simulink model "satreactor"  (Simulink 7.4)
settings: Solver=ode15s  StartTime=0.0  StopTime=0.05  MaxStep=1e-4  RelTol=1e-7  AbsTol=1e-7
libraries: simulink x1

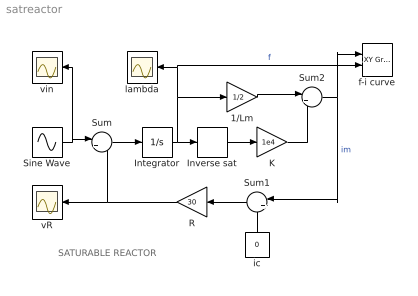
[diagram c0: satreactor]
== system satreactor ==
  note: SATURABLE REACTOR
  1/Lm : Gain  Gain=1/2  ParameterDataType=sfix(16)  ParameterScaling=2^0  OutDataType=sfix(16)  OutScaling=2^0
  Integrator : Integrator
  Inverse sat : DeadZone  LowerValue=-.25  UpperValue=.25
  K : Gain  Gain=1e4  ParameterDataType=sfix(16)  ParameterScaling=2^0  OutDataType=sfix(16)  OutScaling=2^0
  R : Gain  Gain=30  ParameterDataType=sfix(16)  ParameterScaling=2^0  OutDataType=sfix(16)  OutScaling=2^0
  Sine Wave : Sin  Amplitude=120*sqrt(2)  Bias=0  Frequency=2*pi*60  Phase=0  Samples=10  SampleTime=0
  Sum : Sum  Inputs=|+-  OutDataType=sfix(16)  OutScaling=2^0
  Sum1 : Sum  Inputs=|+-  OutDataType=sfix(16)  OutScaling=2^0
  Sum2 : Sum  Inputs=|++  OutDataType=sfix(16)  OutScaling=2^0
  f-i curve : simulink/Sinks/XY Graph  SystemSampleTime=-1  xmin=-0.5  xmax=0.5  ymin=-0.3  ymax=0.3  st=-1
  ic : Constant  Value=0  OutDataType=sfix(16)  OutScaling=2^0
  lambda : Scope
  vR : Scope
  vin : Scope
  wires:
  Inverse sat/1 -> K/1
  Integrator/1 -> Inverse sat/1, 1/Lm/1, f-i curve/2, lambda/1  "f"
  ic/1 -> Sum1/2
  Sum1/1 -> R/1
  Sum/1 -> Integrator/1
  R/1 -> Sum/2, vR/1
  1/Lm/1 -> Sum2/1
  K/1 -> Sum2/2
  Sine Wave/1 -> Sum/1, vin/1
  Sum2/1 -> f-i curve/1, Sum1/1  "im"
